FUNCTION_BLOCK FB53
TITLE =Get Position Is
//*****************************************************************************
//* maxon motor ag
//* R&D
//* all rights reserved
//*****************************************************************************
//* Summary:  Read actual value of position
//*
//* Remarks:
//*
//* Created under: STEP7 REV5.2+SP1
//*****************************************************************************
//* History:
//* 22.04.2004 | INA   first release
//*
//*
//*****************************************************************************
//

AUTHOR:INA
FAMILY:MotionIn
NAME:GetPosIs
VERSION:00.01


VAR_INPUT

Read : BOOL //A rising edge start the command

  NodeID : BYTE //Adress of the maxon device

END_VAR
VAR_OUTPUT
  Done : BOOL //Data valid flag is TRUE if data were available

  Err : BOOL //Error flag is TRUE if an Error has occured, see ErrNo for more details

  ErrNo : DINT //Contains detailed error information

  PositionIs : DINT //Position actual value

END_VAR
VAR
  xEdgeMerker : BOOL //Edge Merker

  xEdgeFlag : BOOL //Edge Flag

  xBusy : BOOL
  xStep : INT
END_VAR

BEGIN

NETWORK
TITLE = Activate the service function
//

// SDO Read "Get Position Is"

       U    #Read
       FP   #xEdgeFlag                   // recognize a positiv edge of the Read signal
       =    #xEdgeMerker                 // and set the xEdgeMerker for one cycle to true

       L    #xStep
       L    0
       ==I
       U    #xEdgeMerker
       SPB  nstp                         // iStep = 1 -> fnc1

       L    #xStep                       // jump list
       SPL  List
       SPA  rdef
       SPA  fnc1
       SPA  fnc2
List  :SPA  rdef

rdef  :NOP  0
       R    #Done                        // reset Done
       R    #Err
       L    0
       T    #xStep                       // iStep = 0
       SPA  end

fnc1  :NOP  0
       CALL FC1
         NodeID:=#NodeID
         Index:=DW#16#00006064
         SubIndex:=DW#16#00000000
         RET_VAL:=#Done
         Err:=#Err
         ErrNo:=#ErrNo

       L    DB219.DBD10
       T    #PositionIs

       SPA  nstp                         // iStep = 1 -> fnc2

fnc2  :NOP  0
       L    0
       T    #xStep
       SPA  end

nstp  :NOP  0
       L    #xStep
       INC            1
       T    #xStep

end   :NOP  0
END_FUNCTION_BLOCK
